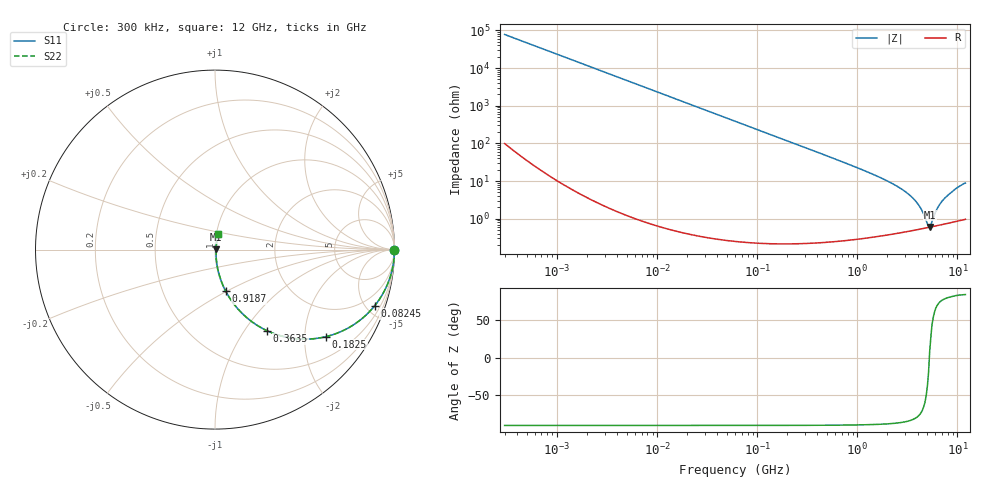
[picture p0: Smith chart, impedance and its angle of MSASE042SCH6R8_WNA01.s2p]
! MSASE042SCH6R8_WNA01  S-PARAMETER MODEL  ( General Type )
! Model Generated by TAIYO YUDEN Corporation (http://www.ty-top.com)
! Version 1.0
! TAIYO YUDEN Control No. 120810
! Copyright(c) 2012 TAIYO YUDEN CO.,LTD. All Rights Reserved.
! Product Description (link to TY-COMPAS)
! https://ds.yuden.co.jp/TYCOMPAS/or/detail?pn=MSASE042SCH6R8BWNA01&u=M
! Products Name : Multilayer Ceramic Capacitors
! Characteristics :
!  Capacitance : 6.8 pF , Rated Voltage : 16V , TCC : CH / C0H
!  Case Size : 0.4 x 0.2 / 0.016 x 0.008 [mm/inch] , Thickness : 0.2 / 0.008 [mm/inch]
!  (Conditions: Temperature = 25 degC , DC Bias Current/Voltage = 0A / 0V)
! External Node Assignments :
!  1  o---| |---o  2
! GND o---------o GND
! Frequency Range : 0.3MHz  -  12000MHz  [ 401 STEP ]
# MHz S RI R 50
! Freq[MHz].  S11 Real  S11 Imag  S21 Real  S21 Imag  S12 Real  S12 Imag  S22 Real  S22 Imag
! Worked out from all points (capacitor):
!   401 points, 300 kHz to 12 GHz, reference 50 ohm
!   read as one part in series: C = 6.81 pF near 316.3 kHz
!   lowest |Z| = 600 mohm at 5.279 GHz (marker M1)
!   series resonance near 5.24 GHz, so ESL is about 140 pH
!   S11 on the Smith chart (normalised r, x): 300 kHz: open; 82.45 MHz: 1.00, -5.66; 182.5 MHz: 1.00, -2.56; 363.5 MHz: 1.00, -1.28; 918.7 MHz: 1.01, -0.49; 12 GHz: 1.02, +0.17
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0.3  1 -0.00128  3.28e-06 0.00128  3.28e-06 0.00128  1 -0.00128
1.769972  0.9999 -0.00758  5.99e-05 0.00758  5.99e-05 0.00758  0.9999 -0.00758
10.44266  0.998 -0.0446  0.00201 0.0446  0.00201 0.0446  0.998 -0.0446
27.10171  0.9867 -0.1145  0.0133 0.1145  0.0133 0.1145  0.9867 -0.1145
60  0.9379 -0.241  0.0621 0.241  0.0621 0.241  0.9379 -0.241
82.45425  0.8889 -0.3138  0.1111 0.3138  0.1111 0.3138  0.8889 -0.3138
182.544  0.62 -0.4846  0.38 0.4846  0.38 0.4846  0.62 -0.4846
353.9943  0.302 -0.4574  0.698 0.4574  0.698 0.4574  0.302 -0.4574
363.4975  0.2909 -0.4524  0.7091 0.4524  0.7091 0.4524  0.2909 -0.4524
570.2811  0.1422 -0.3463  0.8578 0.3463  0.8578 0.3463  0.1422 -0.3463
918.7169  0.0596 -0.2311  0.9404 0.2311  0.9404 0.2311  0.0596 -0.2311
2088.533  0.0124 -0.0927  0.9876 0.0927  0.9876 0.0927  0.0124 -0.0927
2870.14  0.00754 -0.0565  0.9925 0.0565  0.9925 0.0565  0.00754 -0.0565
3642.919  0.00596 -0.033  0.994 0.033  0.994 0.033  0.00596 -0.033
4270.516  0.00562 -0.0185  0.9944 0.0185  0.9944 0.0185  0.00562 -0.0185
5006.236  0.00576 -0.00442  0.9942 0.00442  0.9942 0.00442  0.00576 -0.00442
5278.635  0.0059 0.000838  0.9941 -0.000838  0.9941 -0.000838  0.0059 0.000838
5565.855  0.00611 0.00572  0.9939 -0.00572  0.9939 -0.00572  0.00611 0.00572
6354.153  0.00688 0.0183  0.9931 -0.0183  0.9931 -0.0183  0.00688 0.0183
7064.448  0.00777 0.0286  0.9922 -0.0286  0.9922 -0.0286  0.00777 0.0286
9708.23  0.0123 0.0619  0.9877 -0.0619  0.9877 -0.0619  0.0123 0.0619
12000  0.0169 0.0851  0.9831 -0.0851  0.9831 -0.0851  0.0169 0.0851
